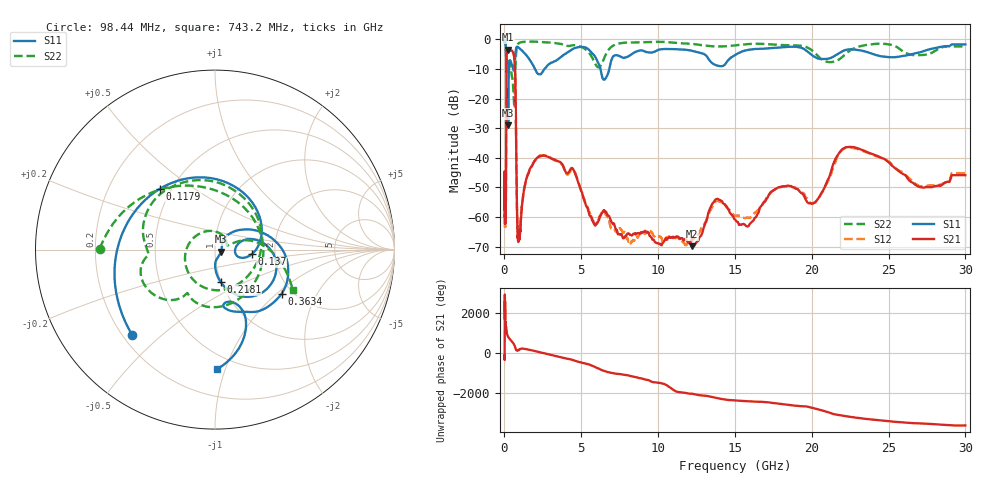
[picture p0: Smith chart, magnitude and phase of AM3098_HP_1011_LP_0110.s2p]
! Date/Time: Thu, Feb 28, 2019 8:43 AM
! Network Analyzer: Agilent Technologies E8364B Rev: A.07.50.67
! Sweep from 0.010 to 30.000 GHz, 1601 Points, Sweep Type: LOG
! Power Supply: 5.023 V, 0.002 A
# Hz S DB R 50
!freq MagS11 AngS11 MagS21 AngS21 MagS12 AngS12 MagS22 AngS22
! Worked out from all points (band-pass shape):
!   1601 points, 10 MHz to 30 GHz, reference 50 ohm
!   highest |S21| = -3.47 dB at 238.7 MHz (marker M1); lowest = -69.9 dB at 12.19 GHz (marker M2)
!   |S21| within 3 dB of the highest: 136.6 MHz to 645.3 MHz (508.7 MHz wide, 130 % of centre)
!   lowest |S11| = -29.1 dB at 239.9 MHz (marker M3), VSWR 1.07, Z = 53.4 - j1.23 ohm
!   |S11| at or under -10 dB: 200.7 MHz to 291.3 MHz (90.55 MHz wide, 36.8 % of centre); 1.993 GHz to 2.601 GHz (607.8 MHz wide, 26.5 % of centre); 6.25 GHz to 6.825 GHz (574.9 MHz wide, 8.79 % of centre)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
!   |S22| runs from -23.1 to -0.5 dB; largest |S21 - S12| = 0.0099
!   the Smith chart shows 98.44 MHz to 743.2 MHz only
!   S11 on the Smith chart (normalised r, x): 98.44 MHz: 0.24, -0.40; 117.9 MHz: 0.43, +0.37; 137 MHz: 1.51, -0.08; 218.1 MHz: 1.00, -0.37; 363.4 MHz: 1.76, -1.08; 743.2 MHz: 0.39, -0.94
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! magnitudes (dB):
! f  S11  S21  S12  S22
! 10 MHz  -0.4  -46.3  -45.7  -0.5
! 38.04 MHz  -0.4  -61.8  -62.5  -0.8
! 98.44 MHz  -3.6  -52.2  -50.3  -3.8
! 117.9 MHz  -6.8  -20.5  -20.6  -10.9
! 137 MHz  -13.7  -6.4  -6.3  -10.3
! 144.7 MHz  -18.4  -5.2  -5.2  -10.8
! 218.1 MHz  -14.8  -3.6  -3.6  -8.2
! 238.7 MHz  -29.0  -3.5  -3.4  -8.6
! 239.9 MHz  -29.1  -3.5  -3.4  -8.6
! 363.4 MHz  -7.0  -3.8  -3.7  -7.8
! 550.5 MHz  -9.8  -4.3  -4.2  -14.7
! 646.1 MHz  -9.6  -6.5  -6.5  -23.0
! 743.2 MHz  -3.5  -25.8  -25.9  -6.2
! 817.4 MHz  -2.4  -58.4  -58.0  -2.3
! 885.5 MHz  -2.6  -68.0  -63.6  -1.5
! 2.084 GHz  -11.0  -40.3  -40.3  -0.8
! 4.48 GHz  -3.1  -43.9  -44.0  -1.9
! 7.926 GHz  -6.0  -66.3  -66.6  -1.1
! 12.19 GHz  -3.8  -69.9  -67.4  -1.5
! 20.2 GHz  -5.9  -55.1  -55.1  -4.6
! 22.56 GHz  -3.3  -36.3  -36.5  -3.5
! 30 GHz  -1.7  -45.9  -45.2  -2.3
